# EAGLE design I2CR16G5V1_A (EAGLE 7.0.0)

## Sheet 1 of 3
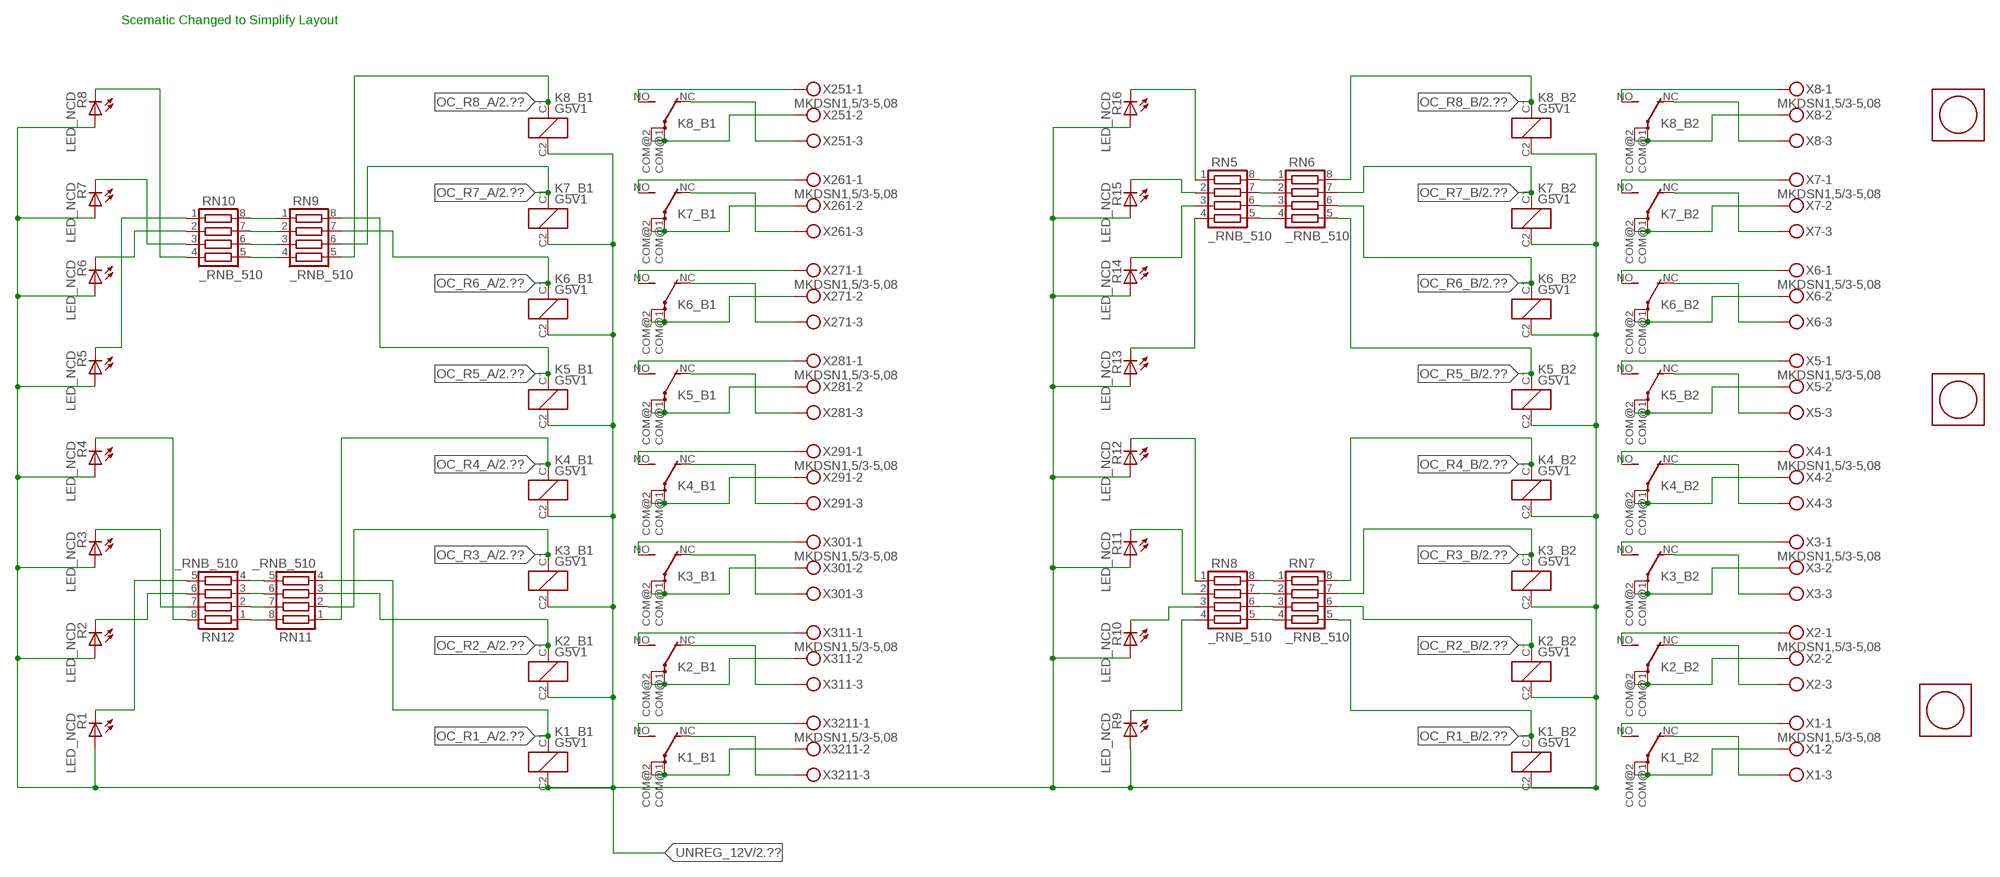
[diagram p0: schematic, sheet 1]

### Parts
K1_B1  G5V1  [G5V1]
K1_B2  G5V1  [G5V1]
K2_B1  G5V1  [G5V1]
K2_B2  G5V1  [G5V1]
K3_B1  G5V1  [G5V1]
K3_B2  G5V1  [G5V1]
K4_B1  G5V1  [G5V1]
K4_B2  G5V1  [G5V1]
K5_B1  G5V1  [G5V1]
K5_B2  G5V1  [G5V1]
K6_B1  G5V1  [G5V1]
K6_B2  G5V1  [G5V1]
K7_B1  G5V1  [G5V1]
K7_B2  G5V1  [G5V1]
K8_B1  G5V1  [G5V1]
K8_B2  G5V1  [G5V1]
R1  LED_NCD  [CHIPLED_0603]
R2  LED_NCD  [CHIPLED_0603]
R3  LED_NCD  [CHIPLED_0603]
R4  LED_NCD  [CHIPLED_0603]
R5  LED_NCD  [CHIPLED_0603]
R6  LED_NCD  [CHIPLED_0603]
R7  LED_NCD  [CHIPLED_0603]
R8  LED_NCD  [CHIPLED_0603]
R9  LED_NCD  [CHIPLED_0603]
R10  LED_NCD  [CHIPLED_0603]
R11  LED_NCD  [CHIPLED_0603]
R12  LED_NCD  [CHIPLED_0603]
R13  LED_NCD  [CHIPLED_0603]
R14  LED_NCD  [CHIPLED_0603]
R15  LED_NCD  [CHIPLED_0603]
R16  LED_NCD  [CHIPLED_0603]
RN5  _RNB_510  [RNB]
RN6  _RNB_510  [RNB]
RN7  _RNB_510  [RNB]
RN8  _RNB_510  [RNB]
RN9  _RNB_510  [RNB]
RN10  _RNB_510  [RNB]
RN11  _RNB_510  [RNB]
RN12  _RNB_510  [RNB]
U$1  PCB_MOUNTING_HOLE  [PCB_MOUNTING_HOLE]
U$2  PCB_MOUNTING_HOLE  [PCB_MOUNTING_HOLE]
U$3  PCB_MOUNTING_HOLE  [PCB_MOUNTING_HOLE]
X1  MKDSN1,5/3-5,08  [MKDSN1,5/3-5,08]
X2  MKDSN1,5/3-5,08  [MKDSN1,5/3-5,08]
X3  MKDSN1,5/3-5,08  [MKDSN1,5/3-5,08]
X4  MKDSN1,5/3-5,08  [MKDSN1,5/3-5,08]
X5  MKDSN1,5/3-5,08  [MKDSN1,5/3-5,08]
X6  MKDSN1,5/3-5,08  [MKDSN1,5/3-5,08]
X7  MKDSN1,5/3-5,08  [MKDSN1,5/3-5,08]
X8  MKDSN1,5/3-5,08  [MKDSN1,5/3-5,08]
X251  MKDSN1,5/3-5,08  [MKDSN1,5/3-5,08]
X261  MKDSN1,5/3-5,08  [MKDSN1,5/3-5,08]
X271  MKDSN1,5/3-5,08  [MKDSN1,5/3-5,08]
X281  MKDSN1,5/3-5,08  [MKDSN1,5/3-5,08]
X291  MKDSN1,5/3-5,08  [MKDSN1,5/3-5,08]
X301  MKDSN1,5/3-5,08  [MKDSN1,5/3-5,08]
X311  MKDSN1,5/3-5,08  [MKDSN1,5/3-5,08]
X3211  MKDSN1,5/3-5,08  [MKDSN1,5/3-5,08]

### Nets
N$1: K8_B2.COM@1(2:P) K8_B2.COM@2(2:P) X8.2
N$2: K8_B2.NC(2:O) X8.3
N$3: K8_B2.NO(2:S) X8.1
N$4: K7_B2.NO(2:S) X7.1
N$5: K6_B2.NO(2:S) X6.1
N$6: K7_B2.NC(2:O) X7.3
N$7: K7_B2.COM@1(2:P) K7_B2.COM@2(2:P) X7.2
N$8: K6_B2.NC(2:O) X6.3
N$10: K4_B2.NO(2:S) X4.1
N$11: K4_B2.NC(2:O) X4.3
N$12: K4_B2.COM@1(2:P) K4_B2.COM@2(2:P) X4.2
N$14: K6_B2.COM@1(2:P) K6_B2.COM@2(2:P) X6.2
N$33: K5_B2.NC(2:O) X5.3
N$34: K5_B2.COM@1(2:P) K5_B2.COM@2(2:P) X5.2
N$35: K5_B2.NO(2:S) X5.1
N$36: K3_B2.NO(2:S) X3.1
N$37: K3_B2.NC(2:O) X3.3
N$38: K3_B2.COM@1(2:P) K3_B2.COM@2(2:P) X3.2
N$39: K2_B2.NO(2:S) X2.1
N$40: K2_B2.NC(2:O) X2.3
N$41: K2_B2.COM@1(2:P) K2_B2.COM@2(2:P) X2.2
N$42: K1_B2.NO(2:S) X1.1
N$43: K1_B2.NC(2:O) X1.3
N$44: K1_B2.COM@1(2:P) K1_B2.COM@2(2:P) X1.2
N$203: K8_B1.COM@1(2:P) K8_B1.COM@2(2:P) X251.2
N$204: K8_B1.NC(2:O) X251.3
N$205: K8_B1.NO(2:S) X251.1
N$206: K7_B1.NO(2:S) X261.1
N$207: K6_B1.NO(2:S) X271.1
N$208: K7_B1.NC(2:O) X261.3
N$209: K7_B1.COM@1(2:P) K7_B1.COM@2(2:P) X261.2
N$210: K6_B1.NC(2:O) X271.3
N$211: K6_B1.COM@1(2:P) K6_B1.COM@2(2:P) X271.2
N$212: K5_B1.NC(2:O) X281.3
N$213: K5_B1.COM@1(2:P) K5_B1.COM@2(2:P) X281.2
N$214: K5_B1.NO(2:S) X281.1
N$215: K4_B1.NO(2:S) X291.1
N$216: K4_B1.NC(2:O) X291.3
N$217: K4_B1.COM@1(2:P) K4_B1.COM@2(2:P) X291.2
N$218: K3_B1.NO(2:S) X301.1
N$219: K3_B1.NC(2:O) X301.3
N$220: K3_B1.COM@1(2:P) K3_B1.COM@2(2:P) X301.2
N$221: K2_B1.NO(2:S) X311.1
N$222: K2_B1.NC(2:O) X311.3
N$223: K2_B1.COM@1(2:P) K2_B1.COM@2(2:P) X311.2
N$224: K1_B1.NO(2:S) X3211.1
N$225: K1_B1.NC(2:O) X3211.3
N$226: K1_B1.COM@1(2:P) K1_B1.COM@2(2:P) X3211.2
N$441: R16.C RN5.1
N$442: RN7.2 RN8.7
N$443: RN7.3 RN8.6
N$444: RN7.4 RN8.5
N$445: R15.C RN5.2
N$447: R13.C RN5.4
N$448: RN5.5 RN6.4
N$449: RN7.1 RN8.8
N$450: R12.C RN8.1
N$451: RN5.6 RN6.3
N$452: R11.C RN8.2
N$453: RN5.7 RN6.2
N$454: RN5.8 RN6.1
N$458: R14.C RN5.3
N$459: R10.C RN8.3
N$463: RN11.5 RN12.4
N$470: R9.C RN8.4
N$473: R1.C RN12.5
N$474: RN11.6 RN12.3
N$475: R2.C RN12.6
N$476: R3.C RN12.7
N$477: RN9.4 RN10.5
N$478: RN9.3 RN10.6
N$479: RN9.2 RN10.7
N$480: RN9.1 RN10.8
N$481: RN11.7 RN12.2
N$482: R5.C RN10.1
N$483: R4.C RN12.8
N$484: R7.C RN10.3
N$485: R8.C RN10.4
N$486: R6.C RN10.2
N$500: RN11.8 RN12.1
OC_R1_A: K1_B1.C1(1:C1) RN11.4 ; also sheet 2
OC_R1_B: K1_B2.C1(1:C1) RN7.5 ; also sheet 2
OC_R2_A: K2_B1.C1(1:C1) RN11.3 ; also sheet 2
OC_R2_B: K2_B2.C1(1:C1) RN7.6 ; also sheet 2
OC_R3_A: K3_B1.C1(1:C1) RN11.2 ; also sheet 2
OC_R3_B: K3_B2.C1(1:C1) RN7.7 ; also sheet 2
OC_R4_A: K4_B1.C1(1:C1) RN11.1 ; also sheet 2
OC_R4_B: K4_B2.C1(1:C1) RN7.8 ; also sheet 2
OC_R5_A: K5_B1.C1(1:C1) RN9.8 ; also sheet 2
OC_R5_B: K5_B2.C1(1:C1) RN6.5 ; also sheet 2
OC_R6_A: K6_B1.C1(1:C1) RN9.7 ; also sheet 2
OC_R6_B: K6_B2.C1(1:C1) RN6.6 ; also sheet 2
OC_R7_A: K7_B1.C1(1:C1) RN9.6 ; also sheet 2
OC_R7_B: K7_B2.C1(1:C1) RN6.7 ; also sheet 2
OC_R8_A: K8_B1.C1(1:C1) RN9.5 ; also sheet 2
OC_R8_B: K8_B2.C1(1:C1) RN6.8 ; also sheet 2
UNREG_12V: K1_B1.C2(1:C2) K1_B2.C2(1:C2) K2_B1.C2(1:C2) K2_B2.C2(1:C2) K3_B1.C2(1:C2) K3_B2.C2(1:C2) K4_B1.C2(1:C2) K4_B2.C2(1:C2) K5_B1.C2(1:C2) K5_B2.C2(1:C2) K6_B1.C2(1:C2) K6_B2.C2(1:C2) K7_B1.C2(1:C2) K7_B2.C2(1:C2) K8_B1.C2(1:C2) K8_B2.C2(1:C2) R1.A R2.A R3.A R4.A R5.A R6.A R7.A R8.A R9.A R10.A R11.A R12.A R13.A R14.A R15.A R16.A ; also sheet 2,3

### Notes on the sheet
- Scematic Changed to Simplify Layout

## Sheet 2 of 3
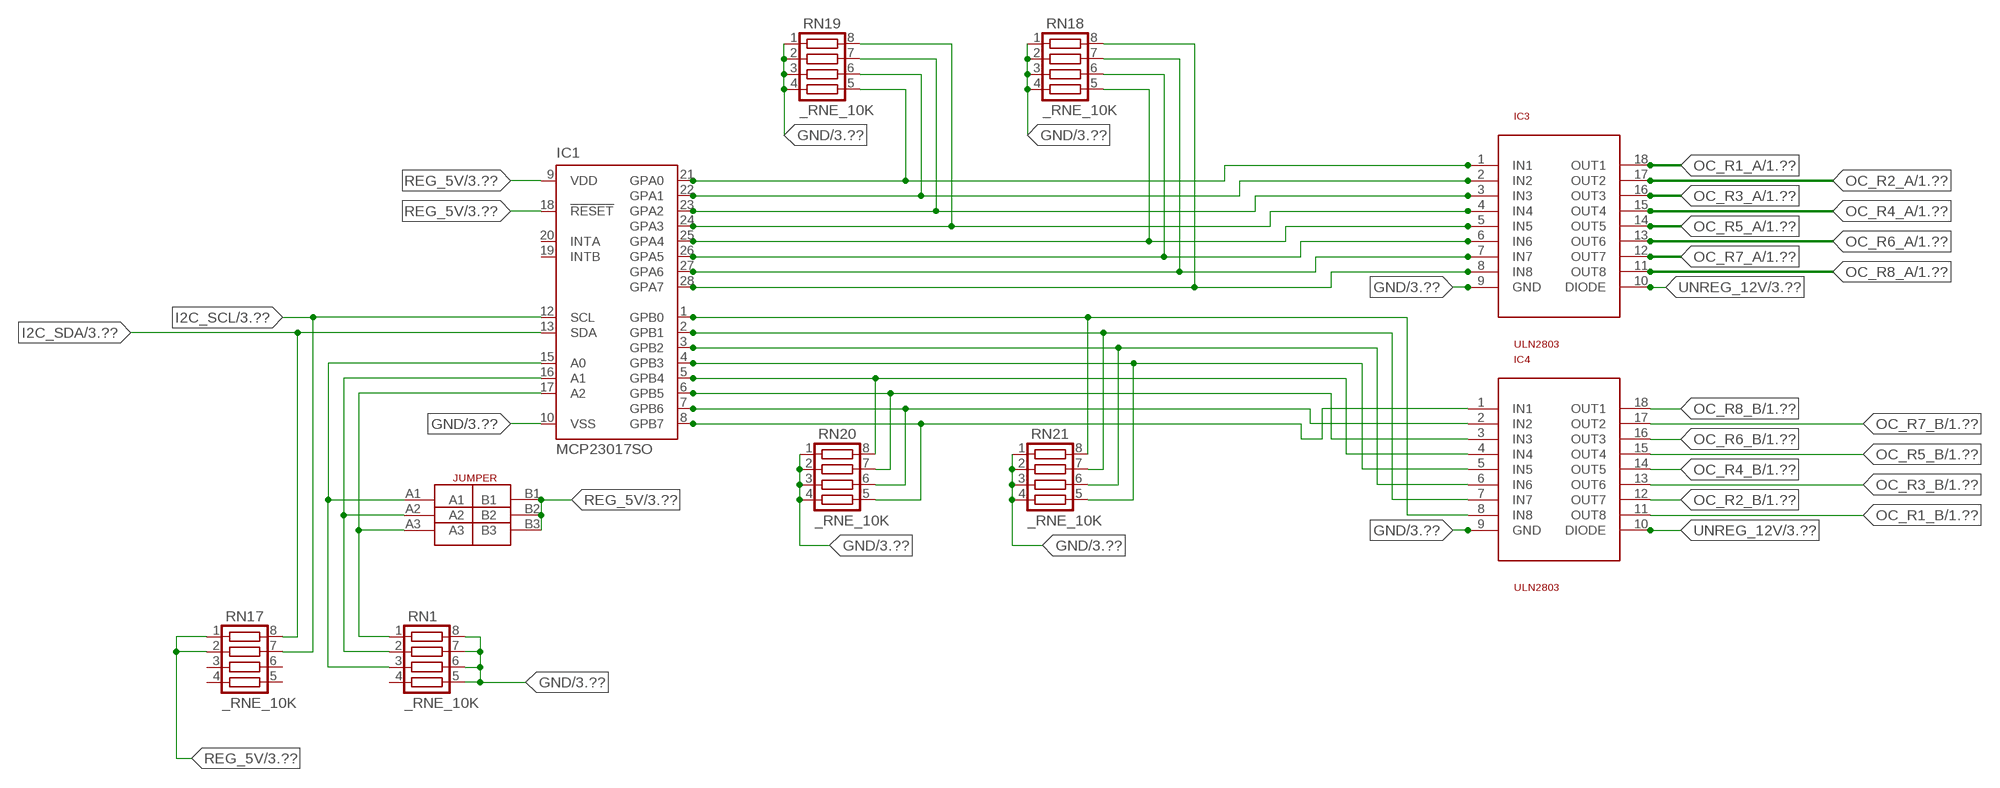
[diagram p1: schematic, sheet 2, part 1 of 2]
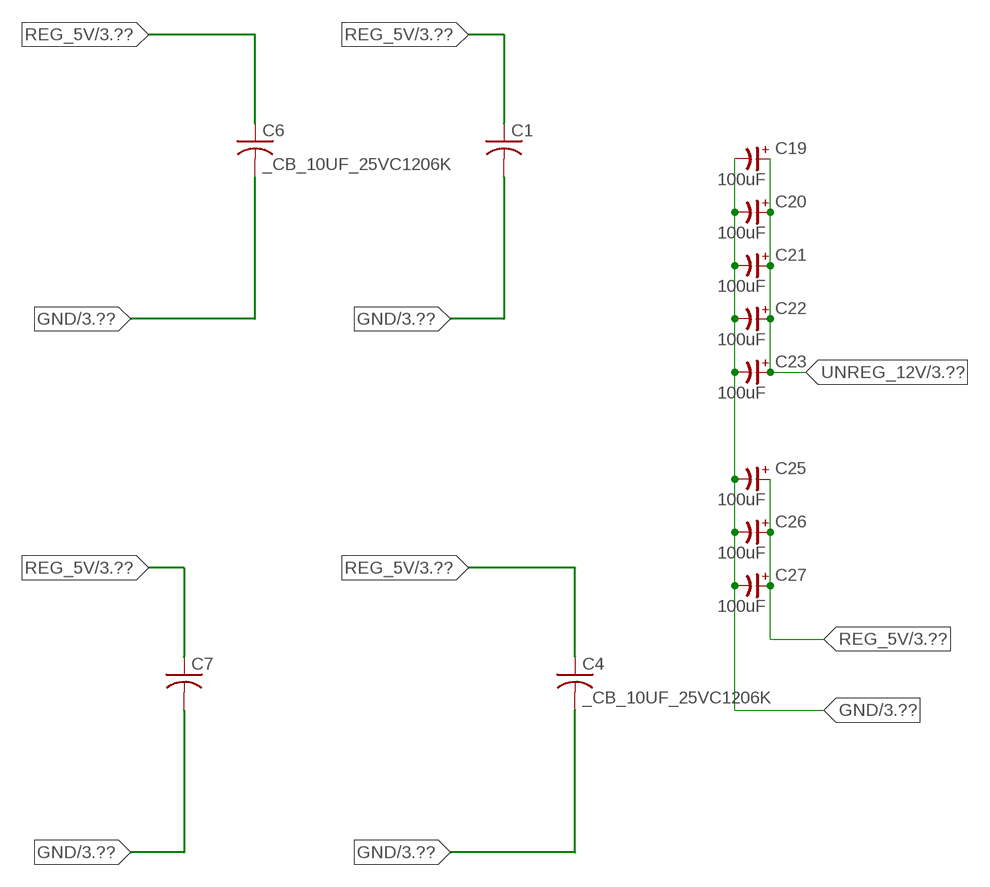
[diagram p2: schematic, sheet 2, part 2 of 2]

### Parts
C1  _CA_.10UF_50VC1206K  [_CA_.1UF_50V]
C4  _CB_10UF_25VC1206K  [_CB_10UF_25V]
C6  _CB_10UF_25VC1206K  [_CB_10UF_25V]
C7  _CA_.10UF_50VC1206K  [_CA_.1UF_50V]
C19  100uF  CP-E-025X060  [E-025X060]
C20  100uF  CP-E-025X060  [E-025X060]
C21  100uF  CP-E-025X060  [E-025X060]
C22  100uF  CP-E-025X060  [E-025X060]
C23  100uF  CP-E-025X060  [E-025X060]
C25  100uF  CP-E-025X060  [E-025X060]
C26  100uF  CP-E-025X060  [E-025X060]
C27  100uF  CP-E-025X060  [E-025X060]
IC1  MCP23017SO  [SO28W]
IC3  ULN2803  [SO18L]
IC4  ULN2803  [SO18L]
JP1  JUMPER_3X2  [JUMPER_3X2]
RN1  _RNE_10K  [RNE]
RN17  _RNE_10K  [RNE]
RN18  _RNE_10K  [RNE]
RN19  _RNE_10K  [RNE]
RN20  _RNE_10K  [RNE]
RN21  _RNE_10K  [RNE]

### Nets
GND: C1.2 C4.2 C6.2 C7.2 C19.- C20.- C21.- C22.- C23.- C25.- C26.- C27.- IC1.10(VSS) IC3.9(GND) IC4.9(GND) RN1.5 RN1.6 RN1.7 RN1.8 RN18.1 RN18.2 RN18.3 RN18.4 RN19.1 RN19.2 RN19.3 RN19.4 RN20.1 RN20.2 RN20.3 RN20.4 RN21.1 RN21.2 RN21.3 RN21.4 ; also sheet 3
I2C_SCL: IC1.12(SCL) RN17.7 ; also sheet 3
I2C_SDA: IC1.13(SDA) RN17.8 ; also sheet 3
N$78: IC1.15(A0) JP1.A1 RN1.3
N$405: IC1.21(GPA0) IC3.1(IN1) RN19.5
N$406: IC1.25(GPA4) IC3.5(IN5) RN18.5
N$407: IC1.26(GPA5) IC3.6(IN6) RN18.6
N$408: IC1.16(A1) JP1.A2 RN1.2
N$409: IC1.22(GPA1) IC3.2(IN2) RN19.6
N$410: IC1.23(GPA2) IC3.3(IN3) RN19.7
N$411: IC1.24(GPA3) IC3.4(IN4) RN19.8
N$416: IC1.1(GPB0) IC4.8(IN8) RN21.8
N$417: IC1.2(GPB1) IC4.7(IN7) RN21.7
N$418: IC1.3(GPB2) IC4.6(IN6) RN21.6
N$419: IC1.4(GPB3) IC4.5(IN5) RN21.5
N$420: IC1.5(GPB4) IC4.4(IN4) RN20.8
N$421: IC1.6(GPB5) IC4.3(IN3) RN20.7
N$422: IC1.7(GPB6) IC4.2(IN2) RN20.6
N$423: IC1.8(GPB7) IC4.1(IN1) RN20.5
N$498: IC1.17(A2) JP1.A3 RN1.1
N$525: IC1.27(GPA6) IC3.7(IN7) RN18.7
N$526: IC1.28(GPA7) IC3.8(IN8) RN18.8
OC_R1_A: IC3.18(OUT1) ; also sheet 1
OC_R1_B: IC4.11(OUT8) ; also sheet 1
OC_R2_A: IC3.17(OUT2) ; also sheet 1
OC_R2_B: IC4.12(OUT7) ; also sheet 1
OC_R3_A: IC3.16(OUT3) ; also sheet 1
OC_R3_B: IC4.13(OUT6) ; also sheet 1
OC_R4_A: IC3.15(OUT4) ; also sheet 1
OC_R4_B: IC4.14(OUT5) ; also sheet 1
OC_R5_A: IC3.14(OUT5) ; also sheet 1
OC_R5_B: IC4.15(OUT4) ; also sheet 1
OC_R6_A: IC3.13(OUT6) ; also sheet 1
OC_R6_B: IC4.16(OUT3) ; also sheet 1
OC_R7_A: IC3.12(OUT7) ; also sheet 1
OC_R7_B: IC4.17(OUT2) ; also sheet 1
OC_R8_A: IC3.11(OUT8) ; also sheet 1
OC_R8_B: IC4.18(OUT1) ; also sheet 1
REG_5V: C1.1 C4.1 C6.1 C7.1 C25.+ C26.+ C27.+ IC1.9(VDD) IC1.18(!RESET) JP1.B1 JP1.B2 JP1.B3 RN17.1 RN17.2 ; also sheet 3
UNREG_12V: C19.+ C20.+ C21.+ C22.+ C23.+ IC3.10(DIODE) IC4.10(DIODE) ; also sheet 1,3
Unconnected: IC1.19(INTB) IC1.20(INTA) RN1.4 RN17.3 RN17.4 RN17.5 RN17.6

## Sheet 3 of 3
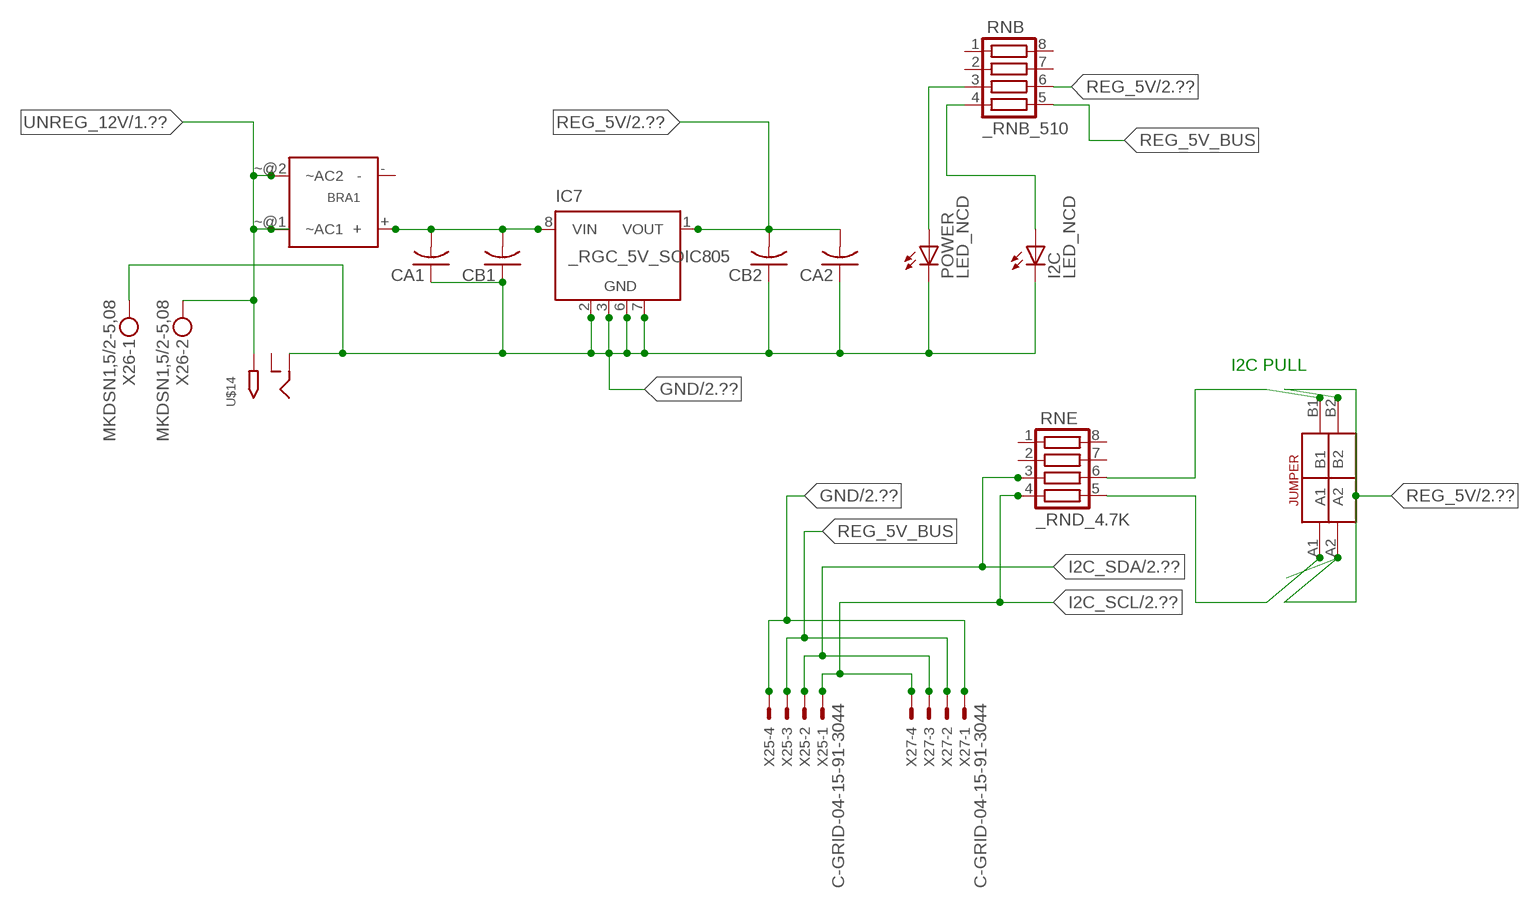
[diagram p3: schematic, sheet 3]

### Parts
BRA1  MB2S_  [MB2S]
CA1  CC1206KRX7R9BB104C1206K  [CC1206KRX7R9BB104]
CA2  CC1206KRX7R9BB104C1206K  [CC1206KRX7R9BB104]
CB1  TMK316F106ZL-TC1206K  [TMK316F106ZL-T]
CB2  TMK316F106ZL-TC1206K  [TMK316F106ZL-T]
I2C  LED_NCD  [CHIPLED_0603]
IC7  _RGC_5V_SOIC805  [_RGC_5V_SOIC8]
POWER  LED_NCD  [CHIPLED_0603]
RNB  _RNB_510  [RNB]
RNE  _RND_4.7K  [RND]
U$14  2.1MMJACK  [PJ-102A]
U$16  JUMPER_2X2  [JUMPER_2X2]
X25  C-GRID-04-15-91-3044  [15-91-04]
X26  MKDSN1,5/2-5,08  [MKDSN1,5/2-5,08]
X27  C-GRID-04-15-91-3044  [15-91-04]

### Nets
GND: CA1.1 CA2.1 CB1.1 CB2.1 I2C.C IC7.2(GND) IC7.3(GND) IC7.6(GND) IC7.7(GND) POWER.C U$14.RING X25.4 X26.1 X27.1 ; also sheet 2
I2C_SCL: RNE.4 X25.1 X27.4 ; also sheet 2
I2C_SDA: RNE.3 X25.2 X27.3 ; also sheet 2
N$513: BRA1.+ CA1.2 CB1.2 IC7.8(VIN)
N$515: POWER.A RNB.3
N$516: I2C.A RNB.4
N$517: RNE.5 U$16.A1
N$518: RNE.6 U$16.B1
REG_5V: CA2.2 CB2.2 IC7.1(VOUT) RNB.6 U$16.A2 U$16.B2 ; also sheet 2
REG_5V_BUS: RNB.5 X25.3 X27.2
UNREG_12V: BRA1.~@1(~AC1) BRA1.~@2(~AC2) U$14.TIP X26.2 ; also sheet 1,2
Unconnected: BRA1.- IC7.4(NC) IC7.5(NC) RNB.1 RNB.2 RNB.7 RNB.8 RNE.1 RNE.2 RNE.7 RNE.8 U$14.RING_SW

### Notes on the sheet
- I2C PULL

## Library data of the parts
BRA1 = NCD_ULTIMATE_LIBRARY:MB2S: Bridge Rectifier BRA MB2S 200V 500ma Digikey MB2S-TPMSTR-ND/MB2S-TP
C1 C7 = NCD_ULTIMATE_LIBRARY:_CA_.10UF_50V: Capacitor .1uF SMT
C4 C6 = NCD_ULTIMATE_LIBRARY:_CB_10UF_25V: Capacitor 10uF SMT
C19-C23 C25-C27 = NCD_ULTIMATE_LIBRARY:CP-: Capacitors All Kinds POLARIZED CAP
CA1 CA2 = NCD_ULTIMATE_LIBRARY:CC1206KRX7R9BB104: Capacitor CA .1uF 50V SMT C1206K CC1206KRX7R9BB104
CB1 CB2 = NCD_ULTIMATE_LIBRARY:TMK316F106ZL-T: Capacitor CB 10uF SMT 1206 TMK316F106ZL-T
I2C POWER R1-R16 = NCD_ULTIMATE_bhaskar:LED_NCD
IC1 = NCD_ULTIMATE_LIBRARY:MCP23017: Semiconductor Port Expander I/O 16-Bit I2C http://ww1.microchip.com/downloads/en/DeviceDoc/21952a.pdf Source: http://ww1.microchip.com/downloads/en/DeviceDoc/21952a.pdf
IC3 IC4 = NCD_ULTIMATE_LIBRARY:ULN2803: Semiconductor 8 O.C. N-Channel Transistor Driver Digikey ULN2803AFWGCELTR-ND/ULN2803AFWG,C,EL
IC7 = NCD_ULTIMATE_LIBRARY:_RGC_5V_SOIC8: Regulator Linear 5V Chip Positive VOLTAGE REGULATOR Digikey 497-7267-2-ND/L78L05CD13TR
JP1 = NCD_ULTIMATE_CONNECTORS:JUMPER_3X2
K1_B1 K1_B2 K2_B1 K2_B2 K3_B1 K3_B2 K4_B1 K4_B2 K5_B1 K5_B2 K6_B1 K6_B2 K7_B1 K7_B2 K8_B1 K8_B2 = NCD_ULTIMATE_LIBRARY:G5V1: RELAY 1 x switch, 0.5 A/125 V AC, 1 A/24 V DC , Omron
RN1 RN17-RN21 = NCD_ULTIMATE_LIBRARY:_RNE_10K: Resistor Array RNE SMT 10K x 4 Single Resistor Source: http://www.ctscorp.com/components/Datasheets/CTSChipArrayDs.pdf Digikey 742C083103JPTR-ND/742C083103JP; OC_FARNELL: unknown; OC_NEWARK: unknown
RN5-RN12 RNB = NCD_ULTIMATE_LIBRARY:_RNB_510: Resistor Array RNB SMT 510 x 4 Single Resistor Source: http://www.ctscorp.com/components/Datasheets/CTSChipArrayDs.pdf Digikey 742C083511JPTR-ND/ 742C083511JP; OC_FARNELL: unknown; OC_NEWARK: unknown
RNE = NCD_ULTIMATE_LIBRARY:_RND_4.7K: Resistor Array RND SMT 4.7K x 4 Single Resistor Source: http://www.ctscorp.com/components/Datasheets/CTSChipArrayDs.pdf Digikey 742C083472JPTR-ND/742C083472JP; OC_FARNELL: unknown; OC_NEWARK: unknown
U$1-U$3 = NCD_ULTIMATE_CONNECTORS:PCB_MOUNTING_HOLE
U$14 = NCD_ULTIMATE_CONNECTORS:2.1MMJACK: 2.1mm x 5.5mm DC jack with internal switch. Digikey part #PJ-102A, 4UCON part #05537 By microbuilder.eu
U$16 = NCD_ULTIMATE_CONNECTORS:JUMPER_2X2
X1-X8 X251 X261 X271 X281 X291 X301 X311 X3211 = NCD_ULTIMATE_CONNECTORS:MKDSN1,5/3-5,08: MKDSN 1,5/ 3-5,08 Printklemme Nennstrom: 13,5 A Nennspannung: 250 V Rastermaß: 5,08 mm Polzahl: 3 Anschlussart: Schraubanschluss Montage: Löten Anschlussrichtung Leiter/Platine: 0 ° Artikelnummer: 1729131 Source: http://eshop.phoenixcontact.com .. 1729131.pdf
X25 X27 = NCD_ULTIMATE_CONNECTORS:C-GRID-04: CONNECTOR 4-Pos I2C wire to board 2.54 mm (0.100") pitch header Digikey WM1342-ND/0015912045; OC_FARNELL: unknown; OC_NEWARK: unknown
X26 = NCD_ULTIMATE_CONNECTORS:MKDSN1,5/2-5,08: MKDSN 1,5/ 2-5,08 Printklemme

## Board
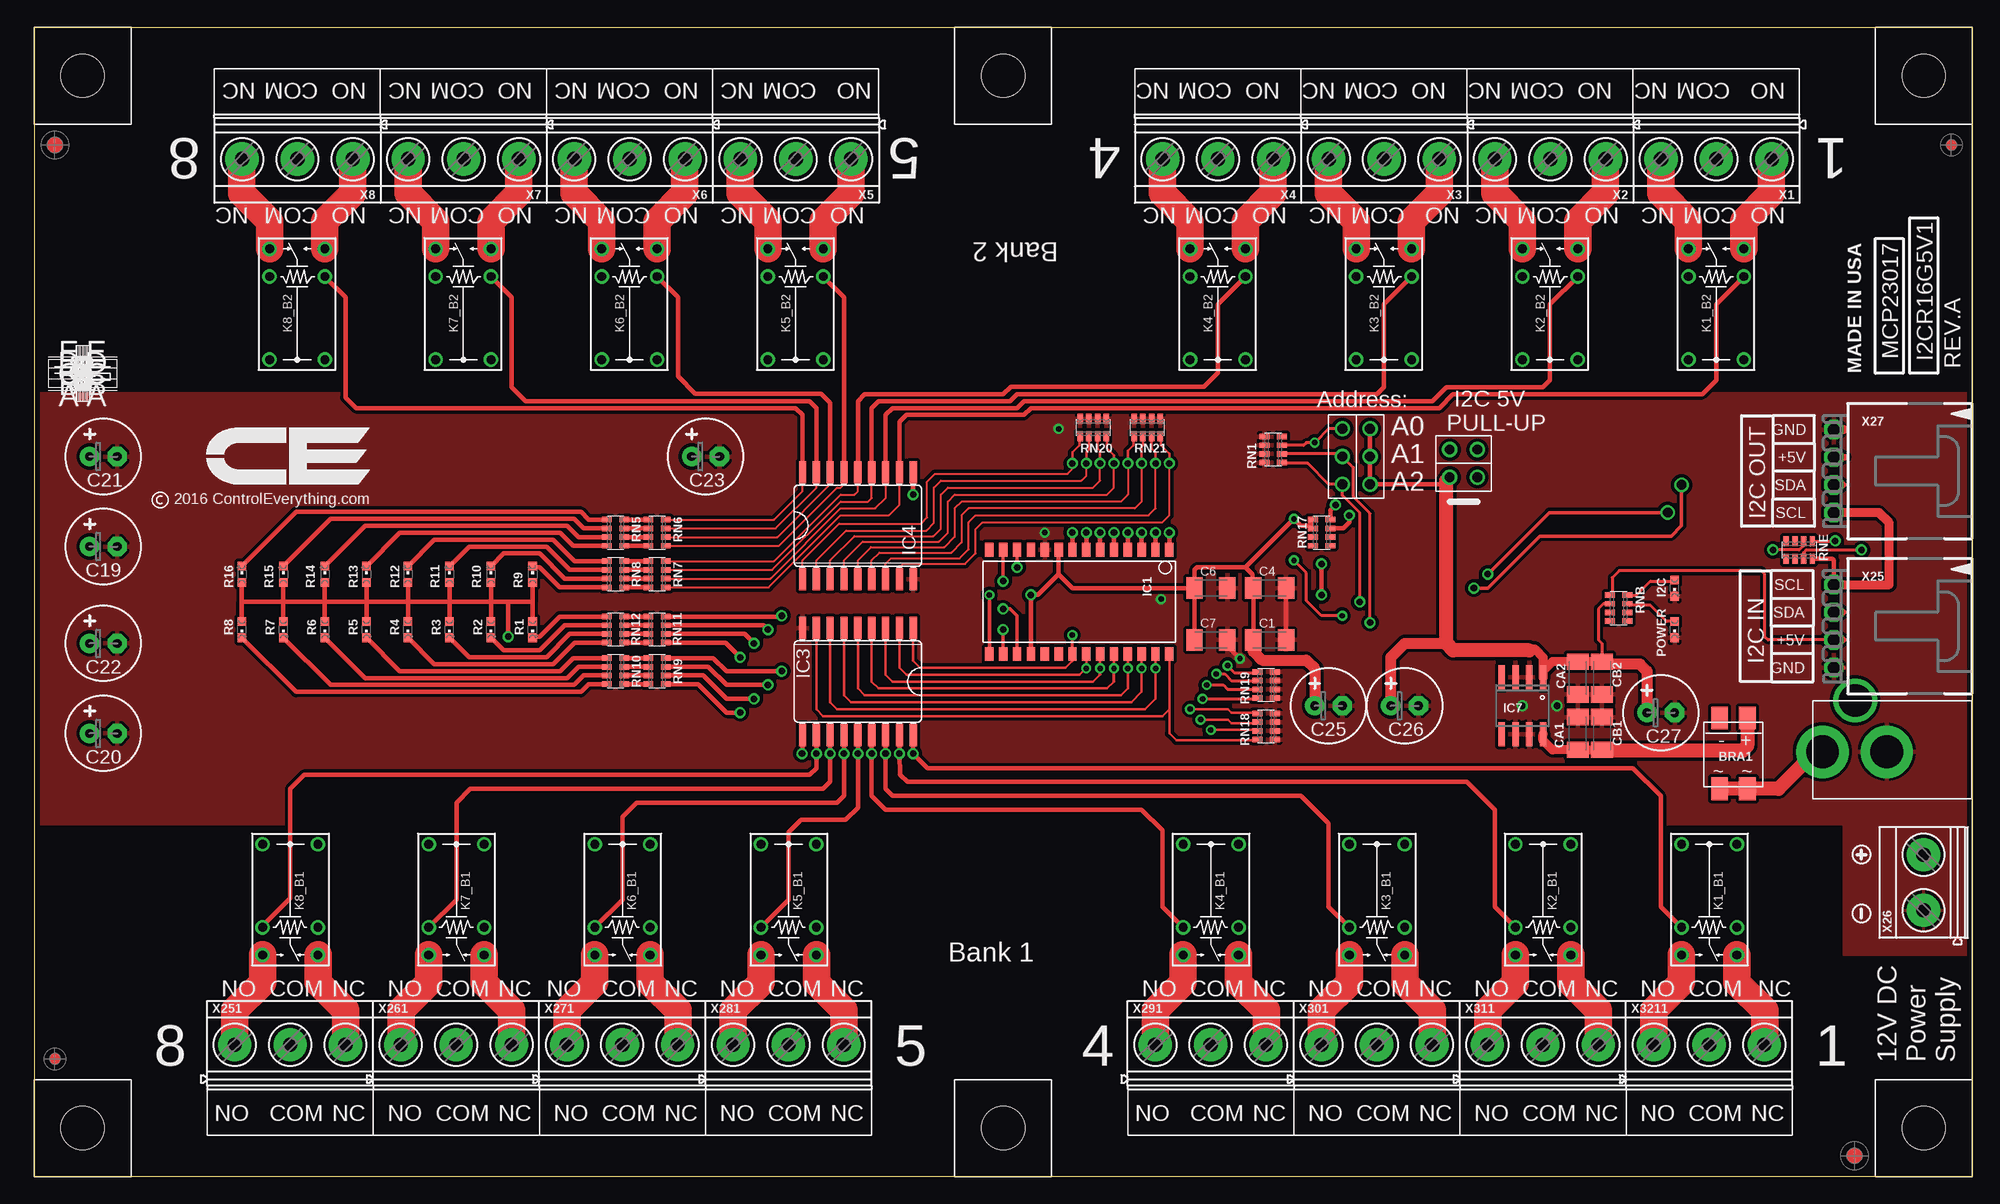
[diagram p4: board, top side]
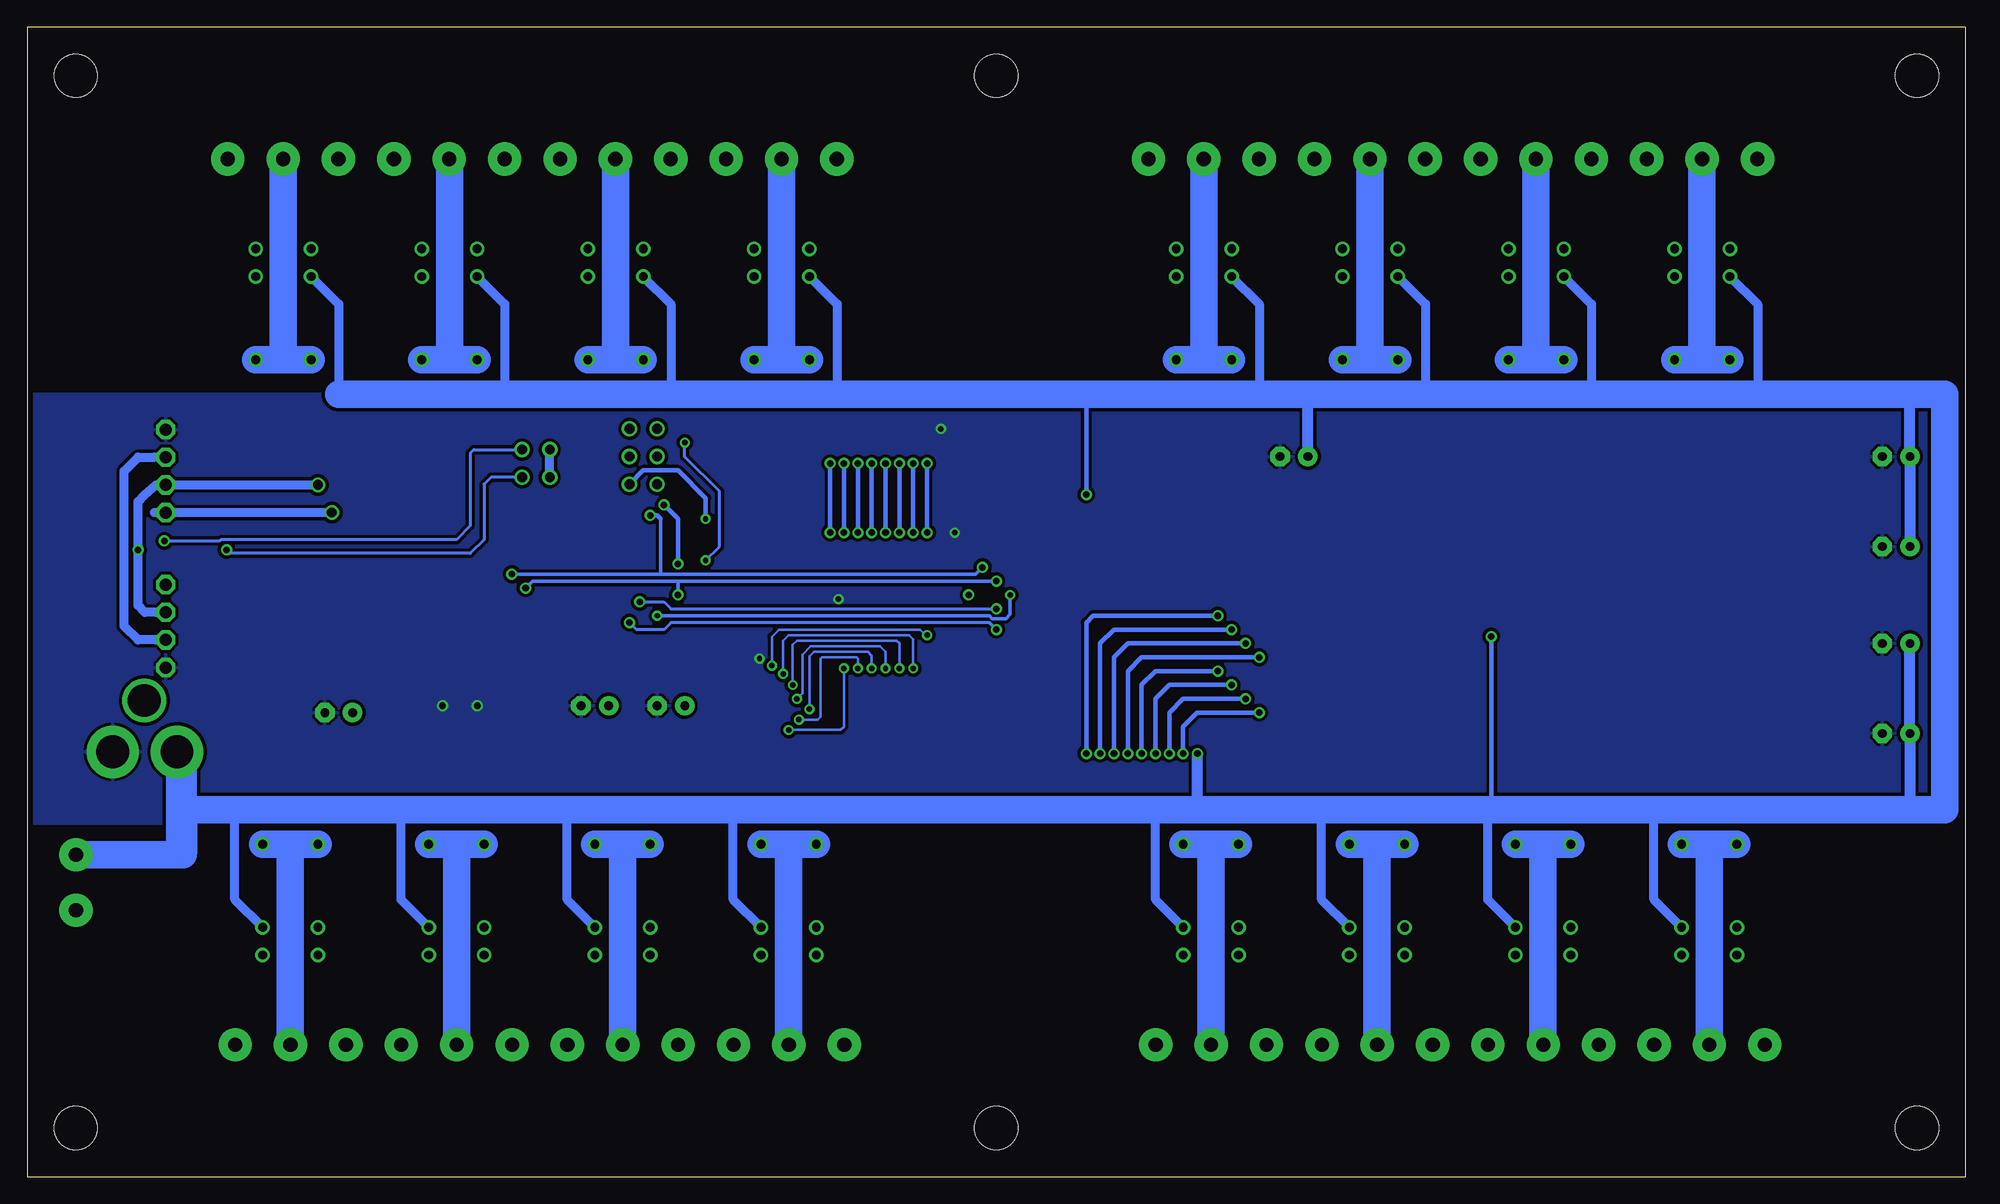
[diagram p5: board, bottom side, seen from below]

Size 177.8 x 105.42 mm. Coordinates in mm from the lower left corner, seen from the top.
Outline: 177.78,105.42 177.78,0
Outline: 177.8,105.42 0,105.42 0,0.01 177.8,0.01
Copper layers (1*16): Top 0.035mm / dielectric 1.5mm / Bottom 0.035mm
Design rules "default *": minimum track width 6mil, minimum drill 12mil, track to track 5mil, track to pad 5mil, pad to pad 5mil, via to via 5mil, smd to smd 5mil, copper to edge 20mil, drill to drill 8mil, minimum pad ring 10mil, minimum via ring 8mil, stop-mask expansion 4mil, vias tented up to drill 0mil, thermal gap 10mil

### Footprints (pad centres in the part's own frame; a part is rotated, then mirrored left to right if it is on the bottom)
MB2S = smd 1.55 x 2.1: + 0,-6.5; - 2.54,-6.5; ~@1 0,0; ~@2 2.54,0
_CA_.1UF_50V = smd 1.5 x 2: 1 -1.5,0; 2 1.5,0
_CB_10UF_25V = smd 1.5 x 2: 1 -1.5,0; 2 1.5,0
E-025X060 = drill 0.813 pad 1.778: + -1.27,0 | drill 0.813 pad 1.778 octagon: - 1.27,0
CC1206KRX7R9BB104 = smd 1.5 x 2: 1 -1.5,0; 2 1.5,0
TMK316F106ZL-T = smd 1.5 x 2: 1 -1.5,0; 2 1.5,0
CHIPLED_0603 = smd 0.8 x 0.8: A 0,-0.75; C 0,0.75
SO28W = smd 0.762 x 1.27: 1 -7.62,-4.78; 2 -6.35,-4.78; 3 -5.08,-4.78; 4 -3.81,-4.78; 5 -2.54,-4.78; 6 -1.27,-4.78; 7 0,-4.78; 8 1.27,-4.78; 9 2.54,-4.78; 10 3.81,-4.78; 11 5.08,-4.78; 12 6.35,-4.78; 13 7.62,-4.78; 14 8.89,-4.78; 15 8.89,4.78; 16 7.62,4.78; 17 6.35,4.78; 18 5.08,4.78; 19 3.81,4.78; 20 2.54,4.78; 21 1.27,4.78; 22 0,4.78; 23 -1.27,4.78; 24 -2.54,4.78; 25 -3.81,4.78; 26 -5.08,4.78; 27 -6.35,4.78; 28 -7.62,4.78
SO18L = smd 0.66 x 2.032: 1 -5.08,-4.902; 2 -3.81,-4.902; 3 -2.54,-4.902; 4 -1.27,-4.902; 5 0,-4.902; 6 1.27,-4.902; 7 2.54,-4.902; 8 3.81,-4.902; 9 5.08,-4.902; 10 5.08,4.902; 11 3.81,4.902; 12 2.54,4.902; 13 1.27,4.902; 14 0,4.902; 15 -1.27,4.902; 16 -2.54,4.902; 17 -3.81,4.902; 18 -5.08,4.902
_RGC_5V_SOIC8 = smd 0.6 x 2.2: 1 -1.905,-2.6; 2 -0.635,-2.6; 3 0.635,-2.6; 4 1.905,-2.6; 5 1.905,2.6; 6 0.635,2.6; 7 -0.635,2.6; 8 -1.905,2.6
JUMPER_3X2 = drill 0.9: A1 0,5.08; A2 0,2.54; A3 0,0; B1 2.54,5.08; B2 2.54,2.54; B3 2.54,0
G5V1 = drill 0.813: C1 -2.54,2.54; C2 -2.54,-2.54; COM@1 5.08,-2.54; COM@2 5.08,2.54; NC -5.08,-2.54; NO -5.08,2.54
RNE = smd 0.5 x 0.9: 1 -1.2,-0.8; 2 -0.4,-0.8; 3 0.4,-0.8; 4 1.2,-0.8; 5 1.2,0.8; 6 0.4,0.8; 7 -0.4,0.8; 8 -1.2,0.8
RNB = smd 0.5 x 0.9: 1 -1.2,-0.8; 2 -0.4,-0.8; 3 0.4,-0.8; 4 1.2,-0.8; 5 1.2,0.8; 6 0.4,0.8; 7 -0.4,0.8; 8 -1.2,0.8
RND = smd 0.5 x 0.9: 1 -1.2,-0.8; 2 -0.4,-0.8; 3 0.4,-0.8; 4 1.2,-0.8; 5 1.2,0.8; 6 0.4,0.8; 7 -0.4,0.8; 8 -1.2,0.8
PCB_MOUNTING_HOLE = hole 3.962: 4.445,4.445
PJ-102A = drill 3 pad 4.8: RING 0.1,-3.39; TIP 0.1,-9.29 | drill 3 pad 3.251: RING_SW -4.6,-6.29
JUMPER_2X2 = drill 0.9: A1 0,2.54; A2 0,0; B1 2.54,2.54; B2 2.54,0
MKDSN1,5/3-5,08 = drill 1.3 pad 3.048: 1 -7.641,0.025; 2 -2.561,0.025; 3 2.519,0.025
15-91-04 = drill 1.1 pad 1.778 octagon: 1 -3.81,-7.62; 2 -1.27,-7.62; 3 1.27,-7.62; 4 3.81,-7.62
MKDSN1,5/2-5,08 = drill 1.3 pad 3.048: 1 -2.561,0.025; 2 2.519,0.025

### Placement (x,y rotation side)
BRA1  157.16,35.57 180 top
C1  113.35,49.23 0 top
C4  113.35,53.99 0 top
C6  107.95,53.99 0 top
C7  107.95,49.23 0 top
C19  6.35,57.8 0 top
C20  6.35,40.65 0 top
C21  6.35,66.05 0 top
C22  6.35,48.91 0 top
C23  61.59,66.05 0 top
C25  118.75,43.19 0 top
C26  125.73,43.19 0 top
C27  149.22,42.56 0 top
CA1  141.6,40.65 270 top
CA2  141.6,45.73 90 top
CB1  143.83,40.65 270 top
CB2  143.83,45.73 90 top
I2C  150.5,53.99 180 top
IC1  96.52,52.72 180 top
IC3  75.56,45.42 180 top
IC4  75.56,59.7 0 top
IC7  136.53,43.19 180 top
JP1  120.02,63.51 0 top
K1_B1  153.67,25.41 90 top
K1_B2  154.31,80.02 270 top
K2_B1  138.43,25.41 90 top
K2_B2  139.06,80.02 270 top
K3_B1  123.19,25.41 90 top
K3_B2  123.83,80.02 270 top
K4_B1  107.95,25.41 90 top
K4_B2  108.58,80.02 270 top
K5_B1  69.22,25.41 90 top
K5_B2  69.85,80.02 270 top
K6_B1  53.98,25.41 90 top
K6_B2  54.61,80.02 270 top
K7_B1  38.73,25.41 90 top
K7_B2  39.37,80.02 270 top
K8_B1  23.5,25.41 90 top
K8_B2  24.13,80.02 270 top
POWER  150.5,50.18 180 top
R1  45.72,50.18 180 top
R2  41.91,50.18 180 top
R3  38.1,50.18 180 top
R4  34.29,50.18 180 top
R5  30.48,50.18 180 top
R6  26.67,50.18 180 top
R7  22.86,50.18 180 top
R8  19.05,50.18 180 top
R9  45.72,55.26 0 top
R10  41.91,55.26 0 top
R11  38.1,55.26 0 top
R12  34.29,55.26 0 top
R13  30.48,55.26 0 top
R14  26.67,55.26 0 top
R15  22.86,55.26 0 top
R16  19.05,55.26 0 top
RN1  113.67,66.69 90 top
RN5  53.34,59.07 270 top
RN6  57.15,59.07 270 top
RN7  57.15,55.26 270 top
RN8  53.34,55.26 270 top
RN9  57.15,46.37 270 top
RN10  53.34,46.37 270 top
RN11  57.15,50.18 90 top
RN12  53.34,50.18 90 top
RN17  118.11,59.07 270 top
RN18  113.03,41.29 90 top
RN19  113.03,45.1 90 top
RN20  97.16,68.72 180 top
RN21  102.11,68.72 180 top
RNB  145.35,52.15 90 top
RNE  161.93,57.48 0 top
U$1  93.34,96.53 90 top
U$2  8.89,96.53 90 top
U$3  177.8,96.53 90 top
U$5  PCB_MOUNTING_HOLE  [PCB_MOUNTING_HOLE]  0,8.9 270 top
U$9  PCB_MOUNTING_HOLE  [PCB_MOUNTING_HOLE]  8.89,96.53 90 top
U$10  PCB_MOUNTING_HOLE  [PCB_MOUNTING_HOLE]  84.45,8.9 270 top
U$11  PCB_MOUNTING_HOLE  [PCB_MOUNTING_HOLE]  168.91,8.9 270 top
U$12  PCB_MOUNTING_HOLE  [PCB_MOUNTING_HOLE]  0,8.9 270 top
U$14  173.35,39.07 270 top
U$15  [VISION_REF15]  167,1.92 90 top
U$16  129.86,66.69 270 top
U$18  [VISION_REF10]  175.9,94.63 90 top
U$21  [ICON_USA]  167.64,73.67 90 top
U$22  [ICON_MINUS]  167.64,24.14 90 top
U$23  [VISION_REF15]  1.91,94.63 90 top
U$24  [ICON_PLUS]  167.64,29.54 0 top
U$28  [VISION_REF10]  1.91,10.81 90 top
X1  151.76,93.36 180 top
X2  136.53,93.36 180 top
X3  121.28,93.36 180 top
X4  106.05,93.36 180 top
X5  67.31,93.36 180 top
X6  52.07,93.36 180 top
X7  36.83,93.36 180 top
X8  21.59,93.36 180 top
X25  172.72,50.5 270 top
X26  173.35,27 90 top
X27  172.72,64.72 270 top
X251  26.04,12.08 0 top
X261  41.27,12.08 0 top
X271  56.52,12.08 0 top
X281  71.75,12.08 0 top
X291  110.49,12.08 0 top
X301  125.73,12.08 0 top
X311  140.97,12.08 0 top
X3211  156.21,12.08 0 top

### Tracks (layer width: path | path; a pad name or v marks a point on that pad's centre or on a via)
GND  (via drill 0.5, 0.6)
  Top 0.406: C1.2 C4.2 | 165.99,46.68 X25.4 | v110.62,47.51 109.86,48.27 109.86,48.82 C7.2
  Top 0.813: X27.1 165.99,68.53
  other vias: 139.7,43.19 136.53,43.19 92.71,59.07 93.98,68.59 103.38,52.97
  pour Top (isolate 0.305): -2.54,32.4 -2.54,71.77 178.12,71.77 178.12,32.4
  pour Top (isolate 0.305): 178.12,20.33 166.05,20.33 166.05,32.4 178.12,32.4
  pour Bottom (isolate 0.305): -1.27,32.4 -1.27,71.77 177.8,71.77 177.8,32.4
I2C_SCL  (via drill 0.6, 0.9)
  Top 0.305: v90.17,55.89 IC1.12 | v149.86,60.91 139,60.91 v133.35,55.26
  Top 0.406: RN17.7 120.1,59.47 120.65,60.02 v120.65,60.65 | X25.1 165.1,56.53 164.97,56.65 163.15,56.65 RNE.4
  Top 0.813: X25.1 170.18,54.3 170.18,59.97 169.24,60.91 X27.4
  Bottom 0.305: v133.35,55.26 119.7,55.26 | 119.7,55.26 90.81,55.26 v90.17,55.89 | 119.7,60.34 119.7,55.26
  Bottom 0.406: v120.65,60.65 120.02,60.65 119.7,60.34
  Bottom 0.813: v149.86,60.91 X27.4 166.12,60.91
I2C_SDA  (via drill 0.6, 0.9)
  Top 0.254: RNE.3 162.32,57.25 162.56,57.48 v167.64,57.48
  Top 0.305: v88.9,54.62 IC1.13 | v151.13,63.45 151.13,59.7 150.18,58.75 138.11,58.75 133.35,53.99 v132.08,53.99
  Top 0.406: RN17.8 118.91,61.14 v119.38,61.61 | v118.11,56.21 v118.11,53.35
  Top 0.61: X27.3 165.99,63.45 | X25.2 165.99,51.76
  Bottom 0.305: 118.11,54.62 131.44,54.62 v132.08,53.99 | 118.11,54.62 v88.9,54.62 | v118.11,53.35 118.11,54.62
  Bottom 0.406: v119.38,61.61 118.11,60.34 v118.11,56.21 | 165.99,51.76 X25.2
  Bottom 0.813: 165.99,51.76 167,51.76 167.64,52.4 v167.64,57.48 167.64,61.93 167,62.56 165.99,63.45 X27.3 v151.13,63.45
N$1
  Bottom 2.54: K8_B2.COM@2 24.13,74.94 | 24.13,74.94 K8_B2.COM@1 | X8.2 24.15,74.96 24.13,74.94
N$2
  Top 2.54: K8_B2.NC 21.59,87.64 19.05,90.18 19.05,93.31 X8.3
N$3
  Top 2.54: K8_B2.NO 26.67,87.64 29.21,90.18 29.21,93.31 X8.1
N$4
  Top 2.54: K7_B2.NO 41.91,87.64 44.45,90.18 44.45,93.31 X7.1
N$5
  Top 2.54: K6_B2.NO 57.15,87.64 59.69,90.18 59.69,93.31 X6.1
N$6
  Top 2.54: K7_B2.NC 36.83,87.64 34.29,90.18 34.29,93.31 X7.3
N$7
  Bottom 2.54: K7_B2.COM@2 39.37,74.94 | 39.37,74.94 K7_B2.COM@1 | X7.2 39.39,74.96 39.37,74.94
N$8
  Top 2.54: K6_B2.NC 52.07,87.64 49.53,90.18 49.53,93.31 X6.3
N$10
  Top 2.54: K4_B2.NO 111.12,87.64 113.67,90.18 113.67,93.31 X4.1
N$11
  Top 2.54: K4_B2.NC 106.05,87.64 103.5,90.18 103.5,93.31 X4.3
N$12
  Bottom 2.54: K4_B2.COM@2 108.58,74.94 | 108.58,74.94 K4_B2.COM@1 | X4.2 108.61,74.96 108.58,74.94
N$14
  Bottom 2.54: K6_B2.COM@2 54.61,74.94 | 54.61,74.94 K6_B2.COM@1 | X6.2 54.63,74.96 54.61,74.94
N$33
  Top 2.54: K5_B2.NC 67.31,87.64 64.77,90.18 64.77,93.31 X5.3
N$34
  Bottom 2.54: K5_B2.COM@2 69.85,74.94 | 69.85,74.94 K5_B2.COM@1 | X5.2 69.87,74.96 69.85,74.94
N$35
  Top 2.54: K5_B2.NO 72.39,87.64 74.93,90.18 74.93,93.31 X5.1
N$36
  Top 2.54: K3_B2.NO 126.36,87.64 128.91,90.18 128.91,93.31 X3.1
N$37
  Top 2.54: K3_B2.NC 121.28,87.64 118.75,90.18 118.75,93.31 X3.3
N$38
  Bottom 2.54: 123.83,74.94 K3_B2.COM@1 | K3_B2.COM@2 123.83,74.94 | 123.83,74.94 123.83,93.31 X3.2
N$39
  Top 2.54: K2_B2.NO 141.6,87.64 144.15,90.18 144.15,93.31 X2.1
N$40
  Top 2.54: K2_B2.NC 136.53,87.64 133.99,90.18 133.99,93.31 X2.3
N$41
  Bottom 2.54: 139.06,74.94 K2_B2.COM@1 | K2_B2.COM@2 139.06,74.94 | 139.06,74.94 139.06,93.31 X2.2
N$42
  Top 2.54: K1_B2.NO 156.84,87.64 159.38,90.18 159.38,93.31 X1.1
N$43
  Top 2.54: K1_B2.NC 151.76,87.64 149.22,90.18 149.22,93.31 X1.3
N$44
  Bottom 2.54: K1_B2.COM@1 154.31,74.94 | K1_B2.COM@2 154.31,74.94 | 154.31,74.94 154.31,93.31 X1.2
N$78  (via drill 0.5)
  Top 0.254: v120.02,51.45 118.11,51.45 116.71,52.84 116.71,55.38 v115.57,56.53 | 114.48,67.07 116.46,67.07 116.71,67.32 v117.47,67.32 118.75,68.59 JP1.A1
  Top 0.305: IC1.15 v87.63,53.35 | 114.48,67.07 RN1.3
  Bottom 0.254: v115.57,56.53 114.3,57.8 114.3,62.88 117.47,66.05 v117.47,67.32
  Bottom 0.305: v87.63,53.35 87.63,51.57 88.01,51.19 89.28,51.19 89.53,51.45 v120.02,51.45
N$203
  Bottom 2.54: 23.5,30.49 K8_B1.COM@2 | K8_B1.COM@1 23.5,30.49 | 23.5,30.49 23.5,12.12 X251.2
N$204
  Top 2.54: K8_B1.NC 26.04,17.79 28.57,15.25 28.57,12.12 X251.3
N$205
  Top 2.54: K8_B1.NO 20.95,17.79 18.41,15.25 18.41,12.12 X251.1
N$206
  Top 2.54: K7_B1.NO 36.2,17.79 33.66,15.25 33.66,12.12 X261.1
N$207
  Top 2.54: K6_B1.NO 51.44,17.79 48.9,15.25 48.9,12.12 X271.1
N$208
  Top 2.54: K7_B1.NC 41.27,17.79 43.81,15.25 43.81,12.12 X261.3
N$209
  Bottom 2.54: K7_B1.COM@2 38.73,30.49 | K7_B1.COM@1 38.73,30.49 | 38.73,30.49 38.73,12.12 X261.2
N$210
  Top 2.54: K6_B1.NC 56.52,17.79 59.05,15.25 59.05,12.12 X271.3
N$211
  Bottom 2.54: K6_B1.COM@2 53.98,30.49 | K6_B1.COM@1 53.98,30.49 | 53.98,30.49 53.98,12.12 X271.2
N$212
  Top 2.54: K5_B1.NC 71.75,17.79 74.3,15.25 74.3,12.12 X281.3
N$213
  Bottom 2.54: K5_B1.COM@2 69.22,30.49 | K5_B1.COM@1 69.22,30.49 | 69.22,30.49 69.22,12.12 X281.2
N$214
  Top 2.54: K5_B1.NO 66.67,17.79 64.14,15.25 64.14,12.12 X281.1
N$215
  Top 2.54: K4_B1.NO 105.41,17.79 102.87,15.25 102.87,12.12 X291.1
N$216
  Top 2.54: K4_B1.NC 110.49,17.79 113.03,15.25 113.03,12.12 X291.3
N$217
  Bottom 2.54: 107.95,30.49 K4_B1.COM@2 | K4_B1.COM@1 107.95,30.49 | 107.95,30.49 107.95,12.12 X291.2
N$218
  Top 2.54: K3_B1.NO 120.65,17.79 118.11,15.25 118.11,12.12 X301.1
N$219
  Top 2.54: K3_B1.NC 125.73,17.79 128.27,15.25 128.27,12.12 X301.3
N$220
  Bottom 2.54: 123.19,30.49 K3_B1.COM@2 | K3_B1.COM@1 123.19,30.49 | 123.19,30.49 123.19,12.12 X301.2
N$221
  Top 2.54: K2_B1.NO 135.89,17.79 133.35,15.25 133.35,12.12 X311.1
N$222
  Top 2.54: K2_B1.NC 140.97,17.79 143.51,15.25 143.51,12.12 X311.3
N$223
  Bottom 2.54: 138.43,30.49 K2_B1.COM@2 | K2_B1.COM@1 138.43,30.49 | 138.43,30.49 138.43,12.12 X311.2
N$224
  Top 2.54: K1_B1.NO 151.13,17.79 148.59,15.25 148.59,12.12 X3211.1
N$225
  Top 2.54: K1_B1.NC 156.21,17.79 158.75,15.25 158.75,12.12 X3211.3
N$226
  Bottom 2.54: 153.67,30.49 K1_B1.COM@2 | K1_B1.COM@1 153.67,30.49 | 153.67,30.49 153.67,12.12 X3211.2
N$405  (via drill 0.5)
  Top 0.229: IC1.21 95.25,47.32 94.61,46.68 81.28,46.68 80.64,47.32 IC3.1
  Top 0.254: 95.25,47.32 v95.25,49.67 | v109.47,46.88 110.11,46.24 112.17,46.24
  Top 0.305: 112.17,46.24 112.23,46.24 RN19.5
  Bottom 0.229: v95.25,49.67 95.25,49.54 95.89,50.18 108.84,50.18 109.47,49.54 v109.47,46.88
N$406  (via drill 0.5)
  Top 0.229: IC1.25 v100.34,46.62 100.33,44.78 99.69,44.15 76.2,44.15 75.56,44.78 IC3.5 | v106.05,42.87 109.54,42.87 109.86,42.56 112.16,42.56 RN18.5
  Bottom 0.229: v100.34,46.62 100.33,47.79 100.69,48.15 105.64,48.15 106.05,47.74 v106.05,42.87
N$407  (via drill 0.5)
  Top 0.229: IC1.26 v101.6,46.62 101.6,44.46 100.65,43.51 74.93,43.51 74.3,44.15 IC3.6 | v107,41.92 109.54,41.92 109.86,41.61 112.15,41.61 RN18.6
  Bottom 0.229: v101.6,46.62 101.6,47.51 101.73,47.64 104.9,47.64 105.03,47.51 105.03,42.18 105.28,41.92 v107,41.92
N$408  (via drill 0.6)
  Top 0.254: v122.56,50.81 122.56,60.85 121.03,62.37 121.03,65.04 JP1.A2 119.76,66.05 119.51,66.31 114.48,66.31 RN1.2
  Top 0.305: v88.9,50.18 IC1.16
  Bottom 0.254: 89.53,50.81 118.75,50.81 119.38,50.18 121.92,50.18 v122.56,50.81
  Bottom 0.305: 89.53,50.81 v88.9,50.18
N$409  (via drill 0.5)
  Top 0.229: IC1.22 96.52,46.68 95.89,46.05 80.01,46.05 79.38,46.68 IC3.2
  Top 0.254: 96.52,46.68 v96.52,46.62 | v108.46,46.11 109.22,46.11 109.86,45.48 112.21,45.48 RN19.6
  Bottom 0.229: v96.52,46.62 96.52,49.29 96.9,49.67 107.95,49.67 108.46,49.16 v108.46,46.11
N$410  (via drill 0.5)
  Top 0.229: IC1.23 97.79,46.05 97.16,45.42 78.74,45.42 78.11,46.05 IC3.3
  Top 0.254: 97.79,46.05 v97.79,46.62 | v107.57,45.1 109.09,45.1 109.47,44.72 112.21,44.72 RN19.7
  Bottom 0.229: v97.79,46.62 97.79,48.91 98.04,49.16 107.19,49.16 107.57,48.78 v107.57,45.1
  Bottom 0.254: 107.82,44.97 v107.57,45.1
N$411  (via drill 0.5)
  Top 0.229: IC1.24 99.06,45.42 98.42,44.78 77.47,44.78 76.83,45.42 IC3.4
  Top 0.254: 99.06,45.42 v99.06,46.62 | v107.19,43.83 112.16,43.83 RN19.8
  Bottom 0.229: v99.06,46.62 99.06,48.15 99.57,48.65 105.92,48.65 106.68,47.89 106.68,44.34 v107.19,43.83
N$416  (via drill 0.6)
  Top 0.203: 79.38,55.89 79.69,56.21 85.41,56.21 86.36,57.16 86.36,59.39 87,60.02 103.5,60.02 104.14,60.65 v104.14,65.42
  Top 0.229: v104.14,65.42 104.14,66.31 103.38,67.07 103.38,67.85 RN21.8
  Top 0.406: v104.14,59.07 IC1.1 | IC4.8 79.38,55.89
  Bottom 0.406: v104.14,65.42 v104.14,59.07
N$417  (via drill 0.6)
  Top 0.203: IC4.7 78.11,56.21 78.61,56.72 84.9,56.72 85.72,57.54 85.72,60.02 86.36,60.65 102.23,60.65 102.87,61.29 v102.87,65.42
  Top 0.229: v102.87,65.42 102.87,66.43 102.49,66.81 102.49,67.9 RN21.7
  Top 0.406: v102.87,59.07 IC1.2
  Bottom 0.406: v102.87,65.42 v102.87,59.07
N$418  (via drill 0.6)
  Top 0.203: IC4.6 76.83,56.53 77.53,57.23 84.14,57.23 85.09,58.18 85.09,60.65 85.72,61.29 100.97,61.29 101.6,61.93 v101.6,65.42
  Top 0.229: v101.6,65.42 101.6,66.94 101.73,67.07 101.73,67.9 RN21.6
  Top 0.406: v101.6,59.07 IC1.3
  Bottom 0.406: v101.6,65.42 v101.6,59.07
N$419  (via drill 0.6)
  Top 0.203: IC4.5 75.56,56.53 76.77,57.73 83.5,57.73 84.45,58.69 84.45,61.29 85.09,61.93 99.69,61.93 100.33,62.56 v100.33,65.42
  Top 0.229: v100.33,65.42 100.33,66.56 100.84,67.07 100.84,67.85 RN21.5
  Top 0.406: v100.33,59.07 IC1.4
  Bottom 0.406: v100.33,59.07 v100.33,65.42
N$420  (via drill 0.6)
  Top 0.203: IC4.4 74.3,56.53 76.01,58.24 83,58.24 83.82,59.07 83.82,61.93 84.45,62.56 98.42,62.56 99.06,63.19 v99.06,65.42
  Top 0.229: v99.06,65.42 99.06,66.18 98.42,66.81 98.42,67.85 RN20.8
  Top 0.406: v99.06,59.07 IC1.5
  Bottom 0.406: v99.06,65.42 v99.06,59.07
N$421  (via drill 0.6)
  Top 0.203: IC4.3 73.03,56.53 75.25,58.75 82.49,58.75 83.19,59.45 83.19,62.56 83.82,63.19 97.16,63.19 97.79,63.83 v97.79,65.42
  Top 0.229: v97.79,65.42 97.79,66.56 97.54,66.81 97.54,67.9 RN20.7
  Top 0.406: v97.79,59.07 IC1.6
  Bottom 0.406: v97.79,65.42 v97.79,59.07
N$422  (via drill 0.6)
  Top 0.203: IC4.2 71.75,56.53 74.49,59.26 81.85,59.26 82.55,59.96 82.55,63.19 83.19,63.83 96.07,63.83 96.52,64.28 v96.52,65.42
  Top 0.229: IC1.7 96.52,57.16 | v96.52,65.42 96.52,66.43 96.77,66.69 96.77,67.9 RN20.6
  Top 0.406: 96.52,65.05 v96.52,65.42 | v96.52,59.07 IC1.7
  Bottom 0.406: v96.52,65.42 v96.52,59.07
N$423  (via drill 0.6)
  Top 0.203: IC4.1 70.48,56.53 73.85,59.89 81.34,59.89 81.92,60.46 81.92,63.76 82.62,64.47 94.8,64.47 95.25,64.91 v95.25,65.42
  Top 0.229: v95.25,65.42 95.25,66.43 95.89,67.07 95.89,67.85 RN20.5
  Top 0.406: v95.25,59.07 IC1.8
  Bottom 0.406: v95.25,59.07 v95.25,65.42
N$441
  Top 0.406: RN5.1 50.87,60.27 50.16,60.97 24.02,60.97 R16.C
N$442
  Top 0.406: RN8.7 RN7.2
N$443
  Top 0.406: RN7.3 RN8.6
N$444
  Top 0.406: RN8.5 RN7.4
N$445
  Top 0.406: RN5.2 50.4,59.47 49.53,60.34 27.19,60.34 R15.C
N$447
  Top 0.406: RN5.4 49.46,57.87 48.26,59.07 33.54,59.07 R13.C
N$448
  Top 0.406: RN5.5 RN6.4
N$449
  Top 0.406: RN7.1 RN8.8
N$450
  Top 0.406: RN8.1 49.6,56.46 47.62,58.43 36.72,58.43 R12.C
N$451
  Top 0.406: RN5.6 RN6.3
N$452
  Top 0.406: RN8.2 49.13,55.66 46.99,57.8 39.89,57.8 R11.C
N$453
  Top 0.406: RN6.2 RN5.7
N$454
  Top 0.406: RN5.8 RN6.1
N$458
  Top 0.406: RN5.3 49.93,58.67 48.9,59.7 30.36,59.7 R14.C
N$459
  Top 0.406: RN8.3 48.66,54.86 46.35,57.16 43.06,57.16 R10.C
N$463
  Top 0.406: RN12.4 RN11.5
N$470
  Top 0.406: RN8.4 48.19,54.06 46.35,55.89 45.84,55.89 R9.C
N$473
  Top 0.406: RN12.5 48.19,51.38 46.35,49.54 45.84,49.54 R1.C
N$474
  Top 0.406: RN11.6 RN12.3
N$475
  Top 0.406: RN12.6 48.66,50.58 46.35,48.27 43.06,48.27 R2.C
N$476
  Top 0.406: RN12.7 49.13,49.78 46.99,47.64 39.89,47.64 R3.C
N$477
  Top 0.406: RN9.4 RN10.5
N$478
  Top 0.406: RN10.6 RN9.3
N$479
  Top 0.406: RN9.2 RN10.7
N$480
  Top 0.406: RN10.8 RN9.1
N$481
  Top 0.406: RN12.2 RN11.7
N$482
  Top 0.406: RN10.1 49.46,47.57 48.26,46.37 33.54,46.37 R5.C
N$483
  Top 0.406: RN12.8 49.6,48.98 47.62,47 36.72,47 R4.C
N$484
  Top 0.406: RN10.3 50.4,45.97 49.53,45.1 27.19,45.1 R7.C
N$485
  Top 0.406: RN10.4 50.87,45.17 50.16,44.46 24.02,44.46 R8.C
N$486
  Top 0.406: RN10.2 49.93,46.77 48.9,45.73 30.36,45.73 R6.C
N$498  (via drill 0.6)
  Top 0.254: v121.6,52.72 121.6,60.91 120.02,62.5 JP1.A3 118.75,63.51 116.84,65.42 114.53,65.42 RN1.1
  Top 0.305: IC1.17 90.17,51.45 89.53,52.08 v88.9,52.08
  Bottom 0.254: v121.6,52.72 119.38,52.72 118.75,52.08 v88.9,52.08
N$500
  Top 0.406: RN11.8 RN12.1
N$513
  Top 0.813: CB1.2 CA1.2 139.29,39.15 138.43,40.02 IC7.8
  Top 1.27: BRA1.+ 157.16,39.51 156.71,39.07 143.91,39.07 CB1.2
N$515
  Top 0.254: POWER.A 149.75,50.93 148.27,52.4 146.3,52.4 RNB.3
  Top 0.305: RNB.3 146.15,52.53
N$516
  Top 0.254: RNB.4 147,53.35 148.27,54.62 150.38,54.62 I2C.A
  Top 0.305: RNB.4
N$517  (via drill 0.6)
  Top 0.254: RNE.5 165.2,58.28 v165.23,58.31
  Bottom 0.254: v165.23,58.31 160.15,58.31 160.02,58.43 138.43,58.43 137.16,59.7 137.16,66.37 136.84,66.69 U$16.A1
N$518  (via drill 0.6)
  Top 0.254: RNE.6 162.32,57.88 161.93,57.48 v159.51,57.48
  Bottom 0.254: U$16.B1 135.25,64.15 135.89,63.51 135.89,58.43 137.16,57.16 159.19,57.16 v159.51,57.48
N$524
  Bottom 0.813: 163.51,29.54 163.83,29.54
  Bottom 2.54: 164.47,38.75 163.83,38.75 163.83,29.54 | 163.51,29.54 163.51,39.07
N$525  (via drill 0.5)
  Top 0.229: IC3.7 73.03,43.51 73.66,42.87 101.92,42.87 102.87,43.83 v102.87,46.62 IC1.27 | v107.95,40.97 111.68,40.97 RN18.7
  Bottom 0.229: v107.95,40.97 103.19,40.97 102.87,41.29 v102.87,46.62
N$526
  Top 0.229: IC1.28 104.14,42.87 | 104.14,42.87 103.5,42.24 72.39,42.24 71.75,42.87 IC3.8 | 104.14,42.87 104.14,40.65 104.78,40.02 112.16,40.02 RN18.8
OC_R1_A  (via drill 0.6)
  Top 0.406: IC3.18 v80.64,38.81 81.98,37.48 146.69,37.48 149.22,34.94 149.22,24.78 K1_B1.C1 | RN11.4 68.51,51.38 v68.58,51.45
  Bottom 0.406: v68.58,51.45 80.01,51.45 80.64,50.81 v80.64,38.81
OC_R1_B
  Top 0.203: RN7.5 67.38,54.06 73.98,60.65 78.42,60.65 79.38,61.61 IC4.11
  Top 0.406: IC4.11 79.38,69.23 80.01,69.86 90.81,69.86 91.44,70.5 128.91,70.5 130.18,71.77 153.03,71.77 154.31,73.04 154.31,80.02 K1_B2.C1
OC_R2_A  (via drill 0.6)
  Top 0.406: RN11.3 66.91,50.58 v67.31,50.18 | IC3.17 v79.38,38.81 79.42,36.87 80.1,36.21 131.44,36.21 133.99,33.67 133.99,24.78 K2_B1.C1
  Bottom 0.406: v67.31,50.18 78.11,50.18 79.38,48.91 v79.38,38.81
OC_R2_B
  Top 0.203: IC4.12 78.11,62.24 77.15,61.29 73.98,61.29 67.55,54.86 RN7.6
  Top 0.406: IC4.12 78.11,69.86 78.74,70.5 90.17,70.5 90.81,71.13 128.27,71.13 129.54,72.4 138.43,72.4 139.06,73.04 139.06,80.02 K2_B2.C1
OC_R3_A  (via drill 0.6)
  Top 0.406: RN11.2 65.17,49.78 v66.04,48.91 | IC3.16 v78.11,38.81 78.11,35.57 78.74,34.94 116.2,34.94 118.75,32.4 118.75,24.78 K3_B1.C1
  Bottom 0.406: v66.04,48.91 76.83,48.91 78.11,47.64 v78.11,38.81
OC_R3_B
  Top 0.203: RN7.7 67.71,55.66 73.98,61.93 76.52,61.93 76.83,62.24 IC4.13
  Top 0.406: IC4.13 76.83,70.5 77.47,71.13 89.53,71.13 90.17,71.77 123.19,71.77 123.83,72.4 123.83,80.02 K3_B2.C1
OC_R4_A  (via drill 0.6)
  Top 0.406: RN11.1 63.43,48.98 v64.77,47.64 | IC3.15 v76.83,38.81 76.83,34.94 78.11,33.67 101.6,33.67 103.5,31.76 103.5,24.78 K4_B1.C1
  Bottom 0.406: v64.77,47.64 75.56,47.64 76.83,46.37 v76.83,38.81
OC_R4_B
  Top 0.203: RN7.8 67.88,56.46 73.98,62.56 75.25,62.56 75.56,62.88 IC4.14
  Top 0.406: IC4.14 75.56,71.13 76.2,71.77 88.9,71.77 89.6,72.47 107.31,72.47 108.58,73.74 108.58,80.02 K4_B2.C1
OC_R5_A  (via drill 0.6)
  Top 0.406: RN9.8 62.3,47.57 63.5,46.37 v68.58,46.37 | IC3.14 v75.56,38.81 75.56,33.86 74.42,32.72 70.36,32.72 69.22,31.57 69.22,25.41 K5_B1.C1
  Bottom 0.406: v68.58,46.37 74.3,46.37 75.56,45.1 v75.56,38.81
OC_R5_B
  Top 0.203: IC4.15 74.3,63.51 73.98,63.19 73.66,63.19 68.33,57.87 RN6.5
  Top 0.406: K5_B2.C1 74.3,80.66 IC4.15
OC_R6_A  (via drill 0.6)
  Top 0.406: RN9.7 61.83,46.77 63.5,45.1 v67.31,45.1 | IC3.13 v74.3,38.81 74.3,34.94 73.66,34.3 55.24,34.3 53.98,33.03 53.98,25.41 K6_B1.C1
  Bottom 0.406: v67.31,45.1 73.03,45.1 74.3,43.83 v74.3,38.81
OC_R6_B
  Top 0.203: RN6.6 68.18,58.67 73.03,63.51 IC4.16
  Top 0.406: IC4.16 73.03,71.01 72.2,71.83 60.62,71.83 59.05,73.4 59.05,80.66 K6_B2.C1
OC_R7_A  (via drill 0.6)
  Top 0.406: RN9.6 61.36,45.97 63.5,43.83 v66.04,43.83 | IC3.12 v73.03,38.81 73.03,36.21 72.39,35.57 40.01,35.57 38.73,34.3 38.73,25.41 K7_B1.C1
  Bottom 0.406: v66.04,43.83 71.75,43.83 73.03,42.56 v73.03,38.81
OC_R7_B
  Top 0.203: RN6.7 68.03,59.47 71.75,63.19 IC4.17
  Top 0.406: IC4.17 71.75,70.5 71.12,71.13 45.09,71.13 43.81,72.4 43.81,80.66 K7_B2.C1
OC_R8_A  (via drill 0.6)
  Top 0.406: RN9.5 60.89,45.17 63.5,42.56 v64.77,42.56 | IC3.11 v71.75,38.81 71.75,37.48 71.12,36.84 24.77,36.84 23.5,35.57 23.5,25.54 20.95,23 K8_B1.C1
  Bottom 0.406: v64.77,42.56 70.48,42.56 71.75,41.29 v71.75,38.81
OC_R8_B
  Top 0.203: RN6.8 67.88,60.27 70.48,62.88 IC4.18
  Top 0.406: IC4.18 70.48,69.86 69.85,70.5 29.53,70.5 28.57,71.45 28.57,80.66 K8_B2.C1
REG_5V  (via drill 0.5, 0.6)
  Top 0.254: RNB.6 143.97,52.55 143.51,52.08 143.51,49.22 143.83,48.91 CB2.2 | 137.03,48.4 130.05,48.4 129.54,48.91
  Top 0.305: RN17.2 117.08,59.47
  Top 0.406: C1.1 C4.1 111.76,54.07 111.76,55.26 111.12,55.89 | C6.1 C7.1 | U$16.B2 129.22,63.51 JP1.B3 JP1.B2 JP1.B1 | 115.64,60.27 v115.57,60.34 | IC1.18 v91.44,53.35 92.08,53.35 93.98,55.26 | 93.98,55.26 IC1.9 | 93.98,55.26 95.25,53.99 C6.1 | C6.1 106.45,55.66 106.68,55.89 111.12,55.89 | 111.12,55.89 v115.57,60.34 | 117.08,59.7 116.2,59.7 v115.57,60.34 | 117.08,59.7 RN17.2 | 117.08,59.7 117.08,60.03 RN17.1
  Top 0.813: CB2.2 CA2.2 139.29,47.23 138.43,46.37 | 138.43,46.37 IC7.1 | 137.03,48.4 137.67,48.4 138.43,47.64 138.43,46.37
  Top 1.016: CB2.2 144.06,47 147.32,47 147.96,46.37 C27.+ | C26.+ 124.46,47.64 125.73,48.91 129.54,48.91 | C1.1 111.85,48.18 112.65,47.38 116.71,47.38 117.47,46.62 C25.+
  Top 1.27: 137.16,48.27 130.18,48.27 129.54,48.91 129.54,63.83 U$16.B2
  Bottom 0.406: v115.57,60.34 115.57,62.24 118.11,64.78 121.28,64.78 JP1.B3
  Bottom 0.813: U$16.B2 U$16.A2
REG_5V_BUS
  Top 0.254: X25.3 159.07,49.22 158.75,49.54 158.75,55.26 158.43,55.57 145.41,55.57 144.78,54.94 144.78,53.35 RNB.5
  Top 0.406: 165.99,49.22 X25.3
  Top 0.61: X25.3 165.74,49.22 165.99,49.22 | X27.2 166.12,65.99
  Bottom 0.406: 165.99,49.22 X25.3 | 166.12,65.99 X27.2
  Bottom 0.813: 165.99,49.22 167.64,49.22 168.91,50.5 168.91,64.72 167.64,65.99 166.12,65.99
UNREG_12V  (via drill 0.6)
  Top 0.305: 45.72,52.72 R1.A
  Top 0.406: IC4.10 v80.64,62.56 | R8.A 19.05,52.72 | R15.A 22.86,52.72 | R6.A 26.67,52.72 | 30.48,52.72 R13.A | R4.A 34.29,52.72 | R3.A 38.1,52.72 | R2.A 41.91,52.72 | R16.A 19.05,52.72 | 19.05,52.72 22.86,52.72 | R7.A 22.86,52.72 | 22.86,52.72 26.67,52.72 | R14.A 26.67,52.72 | 26.67,52.72 30.48,52.72 | R5.A 30.48,52.72 | 30.48,52.72 34.29,52.72 | R12.A 34.29,52.72 | 34.29,52.72 38.1,52.72 | R11.A 38.1,52.72 | 38.1,52.72 41.91,52.72 | R10.A 41.91,52.72 | R9.A 45.72,52.72 | 45.72,50.81 45.72,52.72 | 45.72,52.72 43.5,52.72 | 41.91,52.72 43.5,52.72 | 43.5,52.72 v43.5,49.54 | IC3.10 70.48,39.38 v70.45,38.81
  Top 1.27: U$14.TIP 163.41,38.97 160.02,35.57 BRA1.~@1 BRA1.~@2
  Bottom 0.406: v80.64,62.56 80.64,71.13 80.01,71.77 | v43.5,49.54 43.5,33.67 | 60.39,33.98 60.71,33.67
  Bottom 0.813: K8_B1.C2 28.57,25.41 28.57,33.67 | K7_B1.C2 43.81,25.41 43.81,33.67 | K6_B1.C2 59.05,25.41 59.05,33.67 | K5_B1.C2 74.3,25.41 74.3,33.67 | K4_B1.C2 113.03,25.41 113.03,33.67 | K3_B1.C2 128.27,25.41 128.27,33.67 | K2_B1.C2 143.51,25.41 143.51,33.67 | K1_B1.C2 158.75,25.41 158.75,33.67 | K1_B2.C2 149.22,80.02 149.22,71.77 | K2_B2.C2 133.99,80.02 133.99,71.77 | K3_B2.C2 118.75,80.02 118.75,71.77 | K4_B2.C2 103.5,80.02 103.5,71.77 | K5_B2.C2 64.77,80.02 64.77,71.77 | K6_B2.C2 49.53,80.02 49.53,71.77 | K7_B2.C2 34.29,80.02 34.29,71.77 | K8_B2.C2 19.05,80.02 19.05,71.77
  Bottom 1.016: 60.39,33.98 70.45,33.98 v70.45,38.81 | 61.59,71.13 60.96,71.77 | 2.54,34.3 1.91,33.67 | C23.+ 60.33,71.77 | C22.+ C20.+ 5.08,33.67 | C19.+ C21.+ 5.08,71.77
  Bottom 2.54: 163.83,33.67 163.45,33.29 163.45,29.86 163.79,29.52 X26.2 | 163.83,33.67 158.75,33.67 143.51,33.67 128.27,33.67 113.03,33.67 74.3,33.67 60.71,33.67 59.05,33.67 43.81,33.67 43.5,33.67 28.57,33.67 5.08,33.67 1.91,33.67 1.91,71.77 5.08,71.77 19.05,71.77 34.29,71.77 49.53,71.77 60.33,71.77 60.96,71.77 64.77,71.77 80.01,71.77 103.5,71.77 118.75,71.77 133.99,71.77 149.22,71.77 | 163.22,33.33 163.83,33.67 | 163.83,33.67 163.83,38.73 U$14.TIP

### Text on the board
tNames: NC | COM | NO | NC | COM | NO | NC | COM | NO | NC | COM | NO | NC | COM | NO | NC | COM | NO | NC | COM | NO | NC | COM | NO | 8 | 5 | 4 | 1 | NC | COM | NO | NC | COM | NO | NC | COM | NO | NC | COM | NO | NC | COM | NO | NC | COM | NO | NC | COM | NO | NC | COM | NO | I2CR16G5V1 | Bank 2 | MCP23017 | REV.A | Address: | I2C 5V | PULL-UP | GND | A0 | +5V | A1 | SDA | A2 | 2016 ControlEverything.com | SCL | I2C OUT | SCL | SDA | +5V | I2C IN | GND | Bank 1 | NO | COM | NC | NO | COM | NC | NO | COM | NC | NO | COM | NC | NO | COM | NC | NO | COM | NC | NO | COM | NC | NO | COM | NC | 8 | 5 | 4 | 1 | 12V DC / Power / Supply | NO | COM | NC | NO | COM | NC | NO | COM | NC | NO | COM | NC | NO | COM | NC | NO | COM | NC | NO | COM | NC | NO | COM | NC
